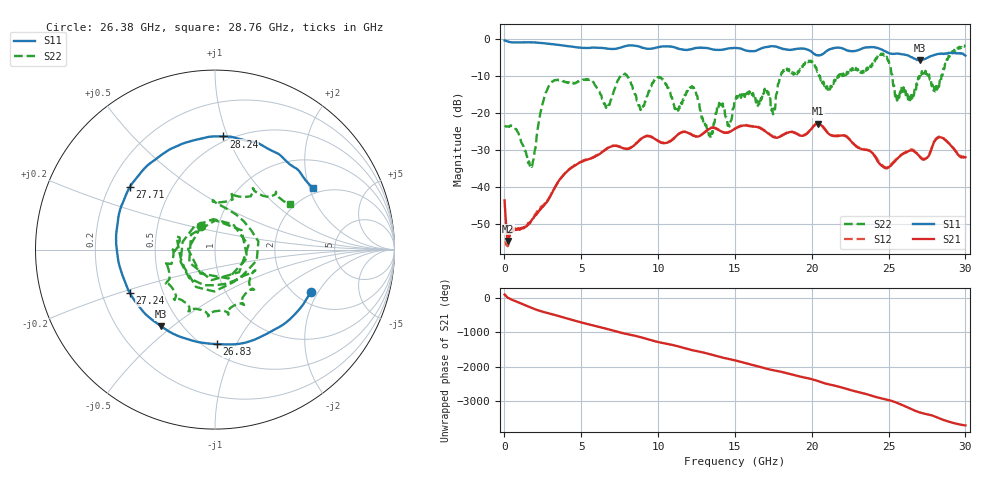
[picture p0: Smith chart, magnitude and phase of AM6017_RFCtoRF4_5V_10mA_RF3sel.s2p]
!Agilent Technologies,E8364B,MY43040894,A.07.50.67
!Agilent E8364B: A.07.50.67
!Date: Tuesday, August 21, 2018 13:30:16
!Correction: S11(Full 2 Port(1,2))
!S21(Full 2 Port(1,2))
!S12(Full 2 Port(1,2))
!S22(Full 2 Port(1,2))
!S2P File: Measurements: S11, S21, S12, S22:
# Hz S  dB  R 50
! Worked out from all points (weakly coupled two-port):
!   1601 points, 10 MHz to 30 GHz, reference 50 ohm
!   highest |S21| = -22.85 dB at 20.38 GHz (marker M1); lowest = -54.5 dB at 234.9 MHz (marker M2)
!   lowest |S11| = -5.7 dB at 27.06 GHz (marker M3), VSWR 3.18, Z = 19.5 - j22.9 ohm
!   |S11| at or under -10 dB: nowhere
!   |S22| runs from -34.5 to -1.6 dB; largest |S21 - S12| = 0.0056
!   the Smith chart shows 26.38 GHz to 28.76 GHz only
!   S11 on the Smith chart (normalised r, x): 26.38 GHz: 2.42, -1.73; 26.83 GHz: 0.58, -0.84; 27.24 GHz: 0.32, -0.22; 27.71 GHz: 0.28, +0.31; 28.24 GHz: 0.46, +0.97; 28.76 GHz: 1.81, +2.11
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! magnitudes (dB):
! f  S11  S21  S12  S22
! 10 MHz  -0.3  -43.5  -55.0  -23.4
! 234.9 MHz  -0.7  -54.5  -55.8  -23.6
! 1.716 GHz  -0.8  -49.3  -49.3  -34.1
! 2.915 GHz  -1.2  -42.9  -42.9  -12.5
! 5.015 GHz  -2.3  -33.1  -33.0  -11.1
! 8.932 GHz  -2.2  -26.8  -26.7  -18.7
! 10.02 GHz  -2.1  -27.6  -27.5  -10.4
! 12.31 GHz  -2.5  -26.1  -26.0  -13.0
! 13.39 GHz  -2.6  -24.1  -24.0  -26.0
! 15.01 GHz  -2.3  -24.2  -24.1  -16.7
! 17.48 GHz  -1.9  -26.4  -26.2  -20.3
! 20.01 GHz  -3.5  -24.0  -23.9  -6.2
! 20.38 GHz  -4.4  -22.8  -22.7  -8.7
! 25.01 GHz  -3.7  -34.6  -34.4  -5.9
! 26.38 GHz  -4.7  -30.1  -29.8  -16.4
! 26.83 GHz  -5.6  -30.8  -30.8  -11.9
! 27.06 GHz  -5.7  -31.9  -31.7  -9.2
! 27.24 GHz  -5.5  -32.5  -32.3  -9.3
! 27.71 GHz  -4.6  -30.6  -30.4  -11.1
! 28.24 GHz  -4.0  -26.6  -26.4  -12.8
! 28.76 GHz  -3.8  -27.5  -27.4  -6.2
! 30 GHz  -4.4  -31.9  -31.9  -1.6
